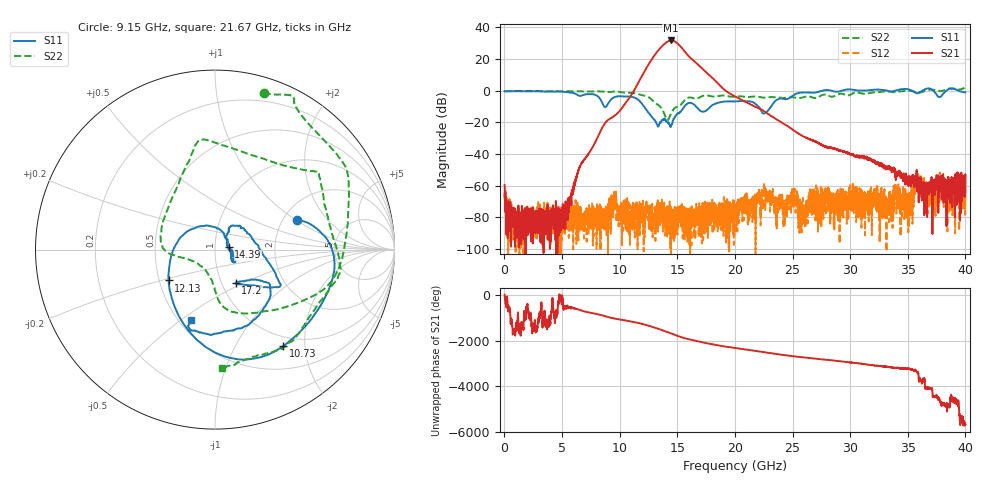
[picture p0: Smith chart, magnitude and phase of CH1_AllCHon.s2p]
!Keysight Technologies,N5245B,MY57181321,A.14.80.03
!Date: Thursday, August 24, 2023 18:02:46
!Correction: S11(C  2-Port  )
!S21(C  2-Port  )
!S12(C  2-Port  )
!S22(C  2-Port  )
!S2P File: Measurements: S11, S21, S12, S22:
# Hz S  RI  R 50
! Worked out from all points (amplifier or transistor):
!   4000 points, 10 MHz to 40 GHz, reference 50 ohm
!   highest |S21| = 31.8 dB at 14.44 GHz (marker M1)
!   |S21| within 3 dB of that: 13.76 GHz to 15.17 GHz (1.412 GHz wide, 9.76 % of centre)
!   unconditionally stable (mu >= 1): start of sweep to 27.54 GHz; 28.42 GHz to 29.24 GHz; 35.38 GHz to 36.25 GHz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
!   at 6.67 GHz: K = 37563.36, MAG = -32.1 dB, |S12| = -79.2 dB
!   at 20.01 GHz: K = 1307.84, MAG = -0.2 dB, |S12| = -71.6 dB
!   at 40 GHz: K = -253554.23, MSG = 2.4 dB, |S12| = -69.3 dB
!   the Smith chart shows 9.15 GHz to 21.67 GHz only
!   S11 on the Smith chart (normalised r, x): 9.15 GHz: 2.37, +1.03; 10.73 GHz: 0.84, -1.59; 12.13 GHz: 0.56, -0.21; 14.39 GHz: 1.16, +0.03; 17.2 GHz: 1.16, -0.46; 21.67 GHz: 0.58, -0.55
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1e7  -0.968 0.0444  0.000939 0.000467  -0.000331 -0.000218  -0.9685 0.0218
6.68e9  0.4116 0.5658  0.00347 0.00357  7.97e-05 5.5e-05  -0.3641 0.8867
9.15e9  0.4568 0.1657  -0.0197 0.1298  6.24e-05 0.000403  0.2712 0.8726
1.073e10  0.3789 -0.5385  0.3238 -0.417  9.38e-05 0.000128  0.6523 0.561
1.213e10  -0.2583 -0.1718  -3.589 1.754  -0.00016 3.47e-05  0.6972 -0.0823
1.283e10  -0.0569 0.1323  6.778 8.042  1.51e-05 7.06e-05  0.3891 -0.3214
1.334e10  0.0693 0.0259  15.31 -10.8  -4.18e-05 8.91e-05  0.0883 -0.3452
1.384e10  0.1119 -0.0586  -16.51 -24.16  9.63e-05 7.53e-05  -0.00918 -0.1965
1.414e10  0.091 -0.0485  -35.62 0.5106  0.000195 6.79e-05  -0.0706 -0.097
1.439e10  0.0759 0.0138  -25.07 29.51  5.63e-06 -8.99e-06  -0.1619 -0.0497
1.444e10  0.0672 0.0321  -19.58 33.62  -4e-06 -7.56e-05  -0.18 -0.0461
1.468e10  0.079 0.1007  10.77 36  6.03e-05 -3.24e-05  -0.2641 -0.0158
1.5e10  0.1317 0.1316  30.38 7.799  -4.59e-05 1.69e-05  -0.3035 0.081
1.526e10  0.2056 0.0652  22.16 -12.98  -4.08e-05 0.00012  -0.2627 0.2275
1.551e10  0.2762 -0.0404  6.882 -18.88  -0.000209 6.4e-05  -0.1892 0.4053
1.612e10  0.3626 -0.2049  -9.503 -5.563  4.67e-05 9.1e-05  -0.064 0.6136
1.72e10  0.1144 -0.1866  0.4137 4.862  1.15e-05 7.93e-05  0.5321 0.4375
2.001e10  0.057 -0.4557  -0.6067 -0.2628  -0.000143 0.000219  0.4898 -0.4315
2.167e10  -0.131 -0.3928  0.0697 0.3164  -0.00017 0.000174  0.0412 -0.6578
2.667e10  -0.5243 -0.7006  -0.00924 0.0262  0.000416 8.87e-05  -0.3841 0.4954
3.334e10  -0.6666 0.7015  0.000772 0.00393  0.000192 0.000187  0.9007 -0.2567
4e10  0.8626 0.2545  0.000222 0.00056  -0.000126 0.000319  0.1269 -1.238
